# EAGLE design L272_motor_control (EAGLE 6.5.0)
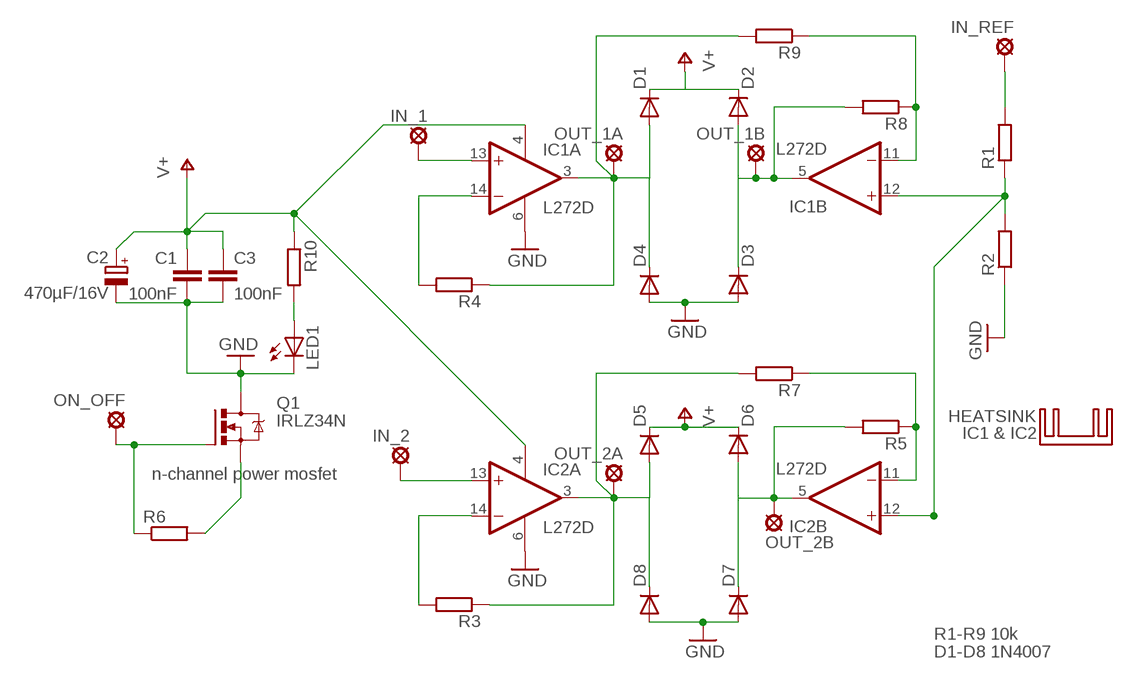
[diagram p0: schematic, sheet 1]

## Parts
C1  100nF  C-EU050-024X044  [C050-024X044]
C2  470µF/16V  CPOL-EUE3.5-8  [E3,5-8]
C3  100nF  C-EU025-024X044  [C025-024X044]
D1  DIODE-DO41-7  [DO41-7]
D2  DIODE-DO41-7  [DO41-7]
D3  DIODE-DO41-7  [DO41-7]
D4  DIODE-DO41-7  [DO41-7]
D5  DIODE-DO41-7  [DO41-7]
D6  DIODE-DO41-7  [DO41-7]
D7  DIODE-DO41-7  [DO41-7]
D8  DIODE-DO41-7  [DO41-7]
HEATSINK  BITMAIN_ANTMINER_HEATSINK  [BITMAIN_ANTMINER_HEATSINK]
IC1  L272D  L272  [SO16]
IC2  L272D  L272  [SO16]
IN_1  SOLPAD_SMALL  [SMALL]
IN_2  SOLPAD_SMALL  [SMALL]
IN_REF  SOLPAD_SMALL  [SMALL]
LED1  LED5MM  [LED5MM]
ON_OFF  SOLPAD_SMALL  [SMALL]
OUT_1A  SOLPAD_SMALL  [SMALL]
OUT_1B  SOLPAD_SMALL  [SMALL]
OUT_2A  SOLPAD_SMALL  [SMALL]
OUT_2B  SOLPAD_SMALL  [SMALL]
Q1  IRLZ34N  IRF740  [TO220BV]
R1  R-EU_R0603  [R0603]
R2  R-EU_R0603  [R0603]
R3  R-EU_0207/10  [0207/10]
R4  R-EU_0207/12  [0207/12]
R5  R-EU_0204/7  [0204/7]
R6  R-EU_0204/7  [0204/7]
R7  R-EU_0207/12  [0207/12]
R8  R-EU_0207/12  [0207/12]
R9  R-EU_0207/12  [0207/12]
R10  R-EU_0204/7  [0204/7]

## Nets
GND: C1.2 C2.- C3.2 D3.A D4.A D7.A D8.A IC1.6(P:GND) IC2.6(P:GND) LED1.K(C) Q1.D R2.1
N$1: IC1.13(A:+IN) IN_1.P$2(MP)
N$2: IC2.14(A:-IN) R3.2
N$3: IC1.12(B:+IN) IC2.12(B:+IN) R1.1 R2.2
N$4: D2.A D3.C IC1.5(B:OUT) OUT_1B.P$2(MP) R8.2
N$5: IN_REF.P$2(MP) R1.2
N$6: LED1.A R10.2
N$7: D1.A D4.C IC1.3(A:OUT) OUT_1A.P$2(MP) R4.1 R9.2
N$8: ON_OFF.P$2(MP) Q1.G R6.1
N$9: D6.A D7.C IC2.5(B:OUT) OUT_2B.P$2(MP) R5.2
N$10: IC1.14(A:-IN) R4.2
N$11: Q1.S R6.2
N$13: IC2.13(A:+IN) IN_2.P$2(MP)
N$14: D5.A D8.C IC2.3(A:OUT) OUT_2A.P$2(MP) R3.1 R7.2
N$15: IC2.11(B:-IN) R5.1 R7.1
N$18: IC1.11(B:-IN) R8.1 R9.1
V+: C1.1 C2.+ C3.1 D1.C D2.C D5.C D6.C IC1.4(P:V+) IC2.4(P:V+) R10.1

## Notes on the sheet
- IC1 & IC2
- n-channel power mosfet
- R1-R9 10k
- D1-D8 1N4007

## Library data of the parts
C1 C3 = rcl:C-EU: CAPACITOR, European symbol
C2 = rcl:CPOL-EU: POLARIZED CAPACITOR, European symbol
D1-D8 = diode:DIODE-: DIODE
HEATSINK = heatsink:BITMAIN_ANTMINER_HEATSINK
IC1 IC2 = linear:L272: OP AMP
IN_1 IN_2 IN_REF ON_OFF OUT_1A OUT_1B OUT_2A OUT_2B = solpad:SOLPAD_SMALL: 1.5MM DIAMETER
LED1 = led:LED: LED
Q1 = transistor-power:IRF740: N-CHANNEL MOS FET
R1-R10 = rcl:R-EU_: RESISTOR, European symbol

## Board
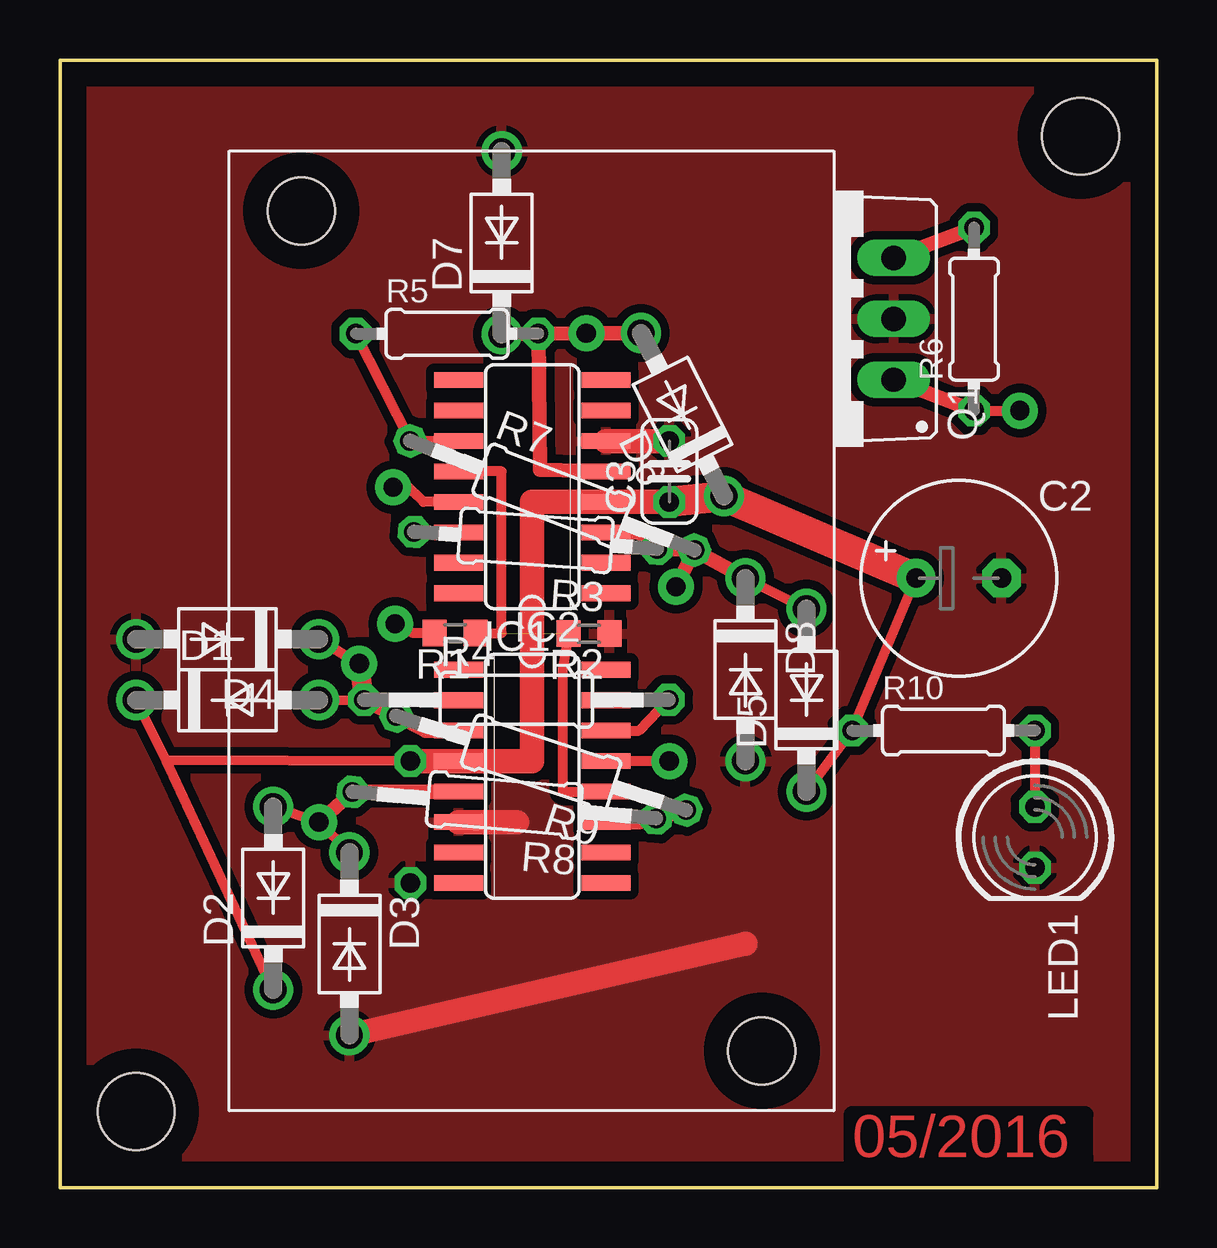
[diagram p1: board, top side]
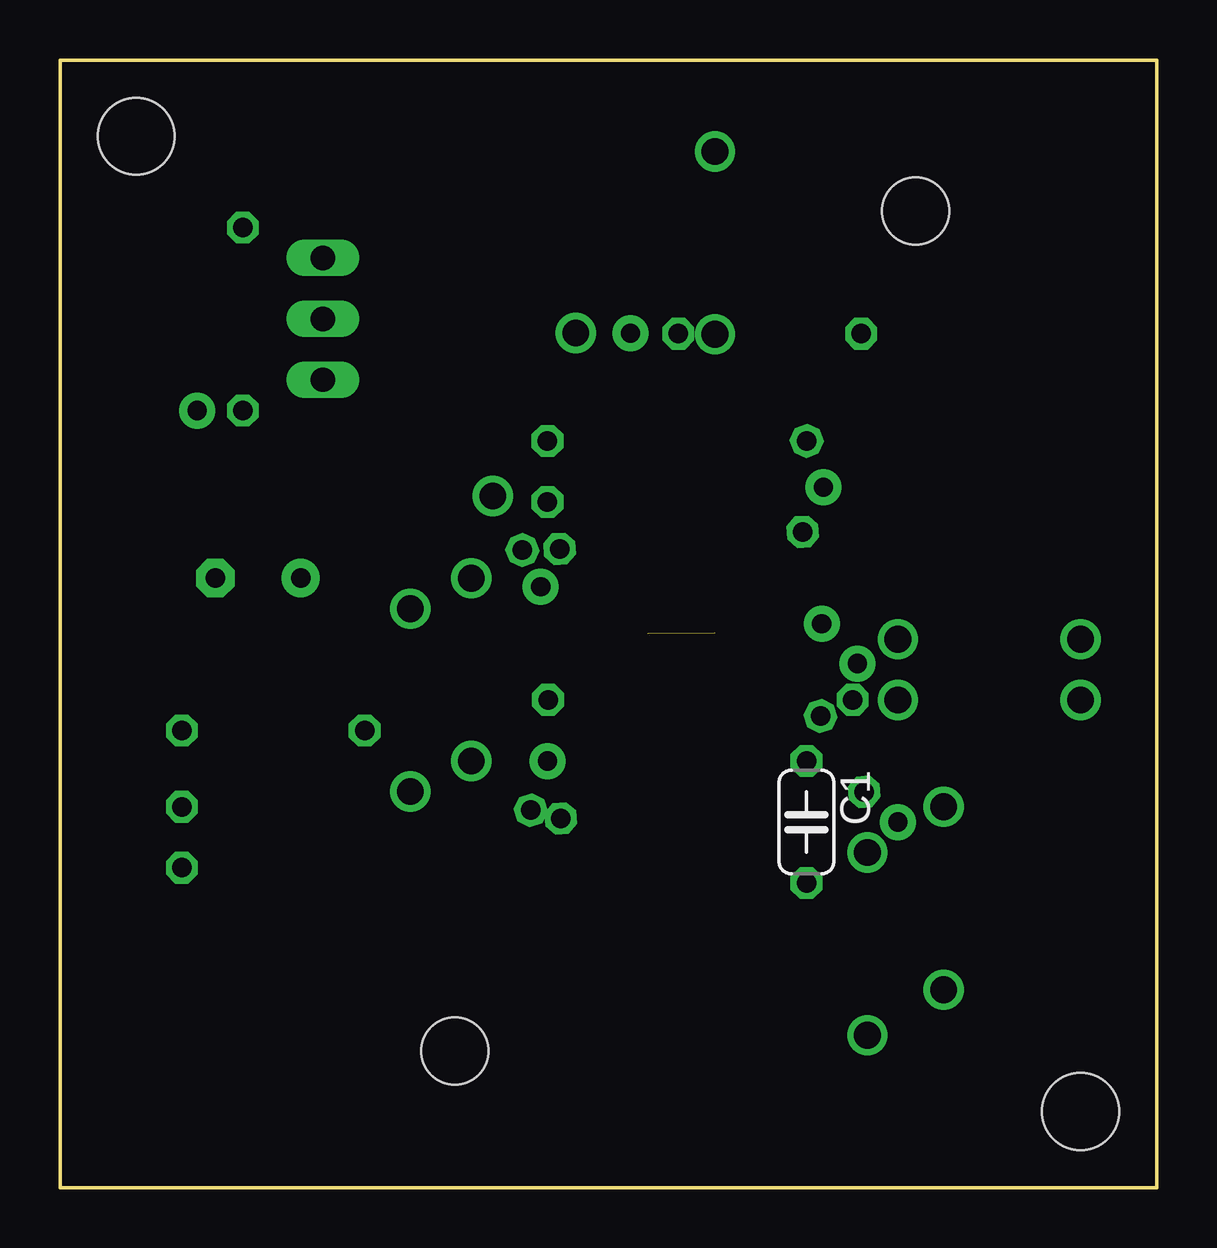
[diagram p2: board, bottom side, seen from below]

Size 45.72 x 46.99 mm. Coordinates in mm from the lower left corner, seen from the top.
Outline: 0,46.99 45.72,46.99 45.72,0 0,0 0,46.99
Copper layers (1*16): Top 0.035mm / dielectric 1.5mm / Bottom 0.035mm
Design rules "default *": minimum track width 10mil, minimum drill 24mil, track to track 14mil, track to pad 14mil, pad to pad 14mil, via to via 14mil, smd to smd 14mil, copper to edge 40mil, drill to drill 8mil, minimum pad ring 10mil, minimum via ring 8mil, stop-mask expansion 4mil, vias tented up to drill 0mil, thermal gap 10mil
Holes 3.2 mm at 42.55,43.82 3.17,3.17

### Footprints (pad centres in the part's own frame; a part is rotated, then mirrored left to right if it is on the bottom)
C050-024X044 = drill 0.813 octagon: 1 -2.54,0; 2 2.54,0
E3,5-8 = drill 0.813 pad 1.6: + -1.778,0 | drill 0.813 pad 1.6 octagon: - 1.778,0
C025-024X044 = drill 0.813 octagon: 1 -1.27,0; 2 1.27,0
DO41-7 = drill 1.118: A 3.81,0; C -3.81,0
BITMAIN_ANTMINER_HEATSINK = hole 2.8: 17.5,9.6; -17.5,-9.6
SO16 = smd 0.66 x 2.032: 1 -4.445,-3.073; 2 -3.175,-3.073; 3 -1.905,-3.073; 4 -0.635,-3.073; 5 0.635,-3.073; 6 1.905,-3.073; 7 3.175,-3.073; 8 4.445,-3.073; 9 4.445,3.073; 10 3.175,3.073; 11 1.905,3.073; 12 0.635,3.073; 13 -0.635,3.073; 14 -1.905,3.073; 15 -3.175,3.073; 16 -4.445,3.073
SMALL = drill 0.8 pad 1.5: P$2 0,0
LED5MM = drill 0.813 octagon: A -1.27,0; K 1.27,0
TO220BV = drill 1.016 long: D 0,-2.54; G -2.54,-2.54; S 2.54,-2.54
R0603 = smd 1 x 1.1: 1 -0.85,0; 2 0.85,0
0207/10 = drill 0.813 octagon: 1 -5.08,0; 2 5.08,0
0207/12 = drill 0.813 octagon: 1 -6.35,0; 2 6.35,0
0204/7 = drill 0.813 octagon: 1 -3.81,0; 2 3.81,0

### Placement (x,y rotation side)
C1  14.61,15.24 270 bottom
C2  37.47,25.4 0 top
C3  25.4,29.84 90 top
D1  6.99,20.32 0 top
D2  8.89,12.06 90 top
D3  12.06,10.16 270 top
D4  6.99,22.86 180 top
D5  31.11,20.32 90 top
D6  25.95,32.22 117 top
D7  18.41,39.37 90 top
D8  28.57,21.59 270 top
HEATSINK  19.66,23.2 90 top
IC1  19.68,17.14 270 top
IC2  19.68,29.21 90 top
IN_1  25.4,17.78 0 top
IN_2  13.89,29.19 0 top
IN_REF  13.97,23.5 0 top
LED1  40.64,14.61 270 top
ON_OFF  40.01,32.38 0 top
OUT_1A  12.48,21.84 0 top
OUT_1B  10.79,15.24 0 top
OUT_2A  25.68,25.04 0 top
OUT_2B  21.94,35.61 0 top
Q1  32.21,36.21 90 top
R1  16.47,23.11 180 top
R2  22.05,23.09 180 top
R3  19.83,26.98 176 top
R4  19.02,20.33 0 top
R5  16.13,35.58 0 top
R6  38.1,36.2 90 top
R7  20.52,28.84 339 top
R8  18.52,15.94 175 top
R9  20.06,17.7 162 top
R10  36.83,19.05 0 top

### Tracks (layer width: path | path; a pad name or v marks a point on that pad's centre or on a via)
GND
  Top 1.016: 28.57,10.16 D3.A | IC1.6 19.05,15.24 | IC2.6 C3.2
  pour Top: 0.64,0.64 45.09,0.64 45.09,46.36 0.64,46.36
N$1
  Top 0.406: IN_1.P$2 IC1.13
N$2
  Top 0.406: R3.2 IC2.14
N$3  (1 unrouted)
  Top 0.406: R2.2 20.95,21.59 20.95,16.51 IC1.12 | R1.1 18.41,23.11 18.41,29.84 IC2.12
N$4
  Top 0.406: D3.C OUT_1B.P$2 D2.A
  Top 0.61: OUT_1B.P$2 R8.2 15.24,16.51 IC1.5
N$5
  Top 0.406: R1.2 14.72,23.11 IN_REF.P$2
N$6
  Top 0.406: R10.2 LED1.A
N$7
  Top 0.406: D4.C OUT_1A.P$2 | D1.A R4.1
  Top 0.61: IC1.3 15.24,19.05 R9.2 R4.1
  Top 0.813: R4.1 OUT_1A.P$2
N$8
  Top 0.406: R6.1 ON_OFF.P$2
  Top 0.61: R6.1 Q1.G
N$9
  Top 0.61: IC2.5 20,29.91 R5.2 | R5.2 D7.C | R5.2 D6.A OUT_2B.P$2
N$10
  Top 0.406: IC1.14 24.13,19.05 R4.2
N$11
  Top 0.61: Q1.S R6.2
N$12  (via drill 0.6 pad 2.8)
  other vias: 29.25,5.7
N$13
  Top 0.406: IC2.13 15.15,28.57 14.88,28.85 14.67,29.06 14.53,29.19 IN_2.P$2
N$14
  Top 0.406: D8.C D5.A
  Top 0.61: IC2.3 24.13,27.3 R3.1 R7.2 | R7.2 OUT_2A.P$2 | R7.2 D8.C
N$15
  Top 0.406: IC2.11 R7.1 R5.1
N$16  (via drill 0.6 pad 2.8)
  other vias: 10.05,40.7
N$18
  Top 0.61: R9.1 R8.1 24.13,15.24 IC1.11
V+
  Top 0.406: D5.C R10.1 C2.+ | D2.C 4.43,17.82 | 4.43,17.82 D1.C | C1.1 4.43,17.82
  Top 1.016: C1.1 IC1.4 19.68,17.78 19.68,28.57 IC2.4 C3.1
  Top 1.27: C2.+ D6.C C3.1

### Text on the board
Top: 05/2016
